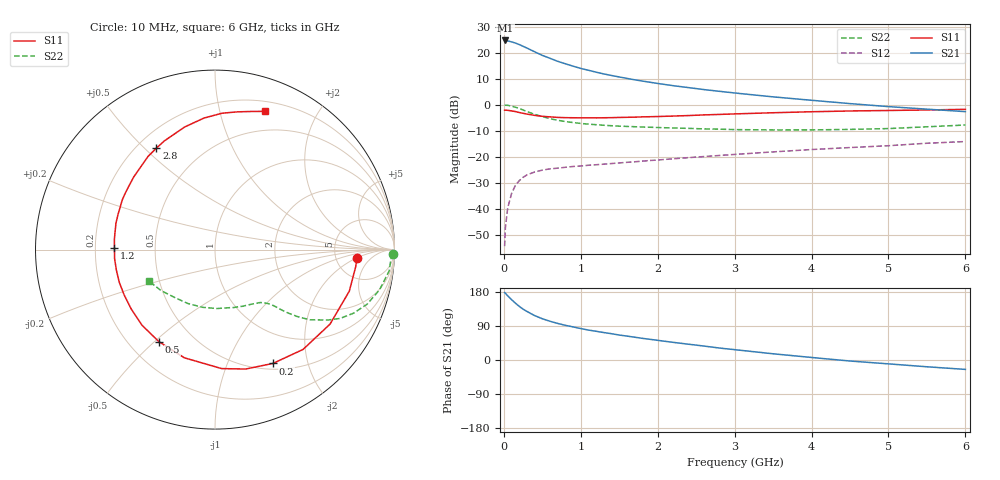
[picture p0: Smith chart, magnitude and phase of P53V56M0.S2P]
! SIEMENS Small Signal Semiconductors
! BFP183
! Si NPN RF Bipolar Junction Transistor in SOT143
! VCE = 3.5 V  IC = 6 mA
! Common Emitter S-Parameters:  March  1996
# GHz  S  MA  R  50
!  f  S11  S21  S12  S22
! GHz  MAG  ANG  MAG  ANG  MAG  ANG  MAG  ANG
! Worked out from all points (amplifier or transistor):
!   36 points, 10 MHz to 6 GHz, reference 50 ohm
!   highest |S21| = 24.8 dB at 20 MHz (marker M1)
!   |S21| within 3 dB of that: start of sweep to 305.8 MHz
!   unconditionally stable (mu >= 1): 1.468 GHz to 5.659 GHz
!   at 250 MHz: K = 0.23, MSG = 25.2 dB, |S12| = -27.9 dB
!   at 1.4 GHz: K = 0.98, MSG = 17.0 dB, |S12| = -22.6 dB
!   at 6 GHz: K = 0.95, MSG = 5.8 dB, |S12| = -14.1 dB
!   lowest NFmin = 1.20 dB at 450 MHz
!   S11 on the Smith chart (normalised r, x): 10 MHz: 8.08, -2.03; 200 MHz: 0.57, -1.47; 500 MHz: 0.32, -0.52; 1.2 GHz: 0.28, +0.01; 2.8 GHz: 0.28, +0.54; 6 GHz: 0.30, +1.38
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0.01  0.7917 -3.4  17.2 178.0  0.0019 86.7  0.9921 -1.4
0.02  0.79 -6.8  17.34 176.1  0.0043 87.7  0.9821 -2.8
0.05  0.7833 -17.2  16.98 169.4  0.0103 84.5  0.9776 -7.0
0.1  0.7637 -32.9  16.3 159.4  0.0195 73.0  0.9434 -13.8
0.15  0.7416 -48.6  15.46 150.0  0.0282 66.0  0.8999 -19.8
0.2  0.7116 -63.0  14.48 141.6  0.0346 59.9  0.8487 -24.7
0.25  0.6871 -75.6  13.38 134.2  0.0402 54.9  0.7959 -28.8
0.3  0.664 -86.8  12.39 128.2  0.0447 51.0  0.7422 -31.9
0.4  0.6265 -105.8  10.49 117.2  0.0509 44.4  0.6578 -36.5
0.5  0.6007 -121.3  8.947 108.9  0.0553 40.1  0.5916 -39.1
0.6  0.5857 -133.9  7.859 102.2  0.0585 37.6  0.5407 -40.9
0.7  0.5722 -144.6  6.878 96.5  0.0603 36.1  0.5034 -42.1
0.9  0.5637 -161.2  5.548 87.3  0.065 33.9  0.4554 -43.6
1.1  0.5617 -174.8  4.622 79.0  0.0687 33.2  0.4244 -45.3
1.2  0.5603 179.2  4.247 75.8  0.0702 33.2  0.4142 -46.2
1.7  0.5789 155.9  3.03 60.2  0.08 34.2  0.3789 -52.1
2.2  0.6074 138.2  2.338 46.6  0.0914 34.7  0.3579 -59.8
2.8  0.6529 120.0  1.821 31.6  0.1057 33.9  0.3399 -71.7
3.5  0.7037 103.9  1.422 16.4  0.1241 32.1  0.3286 -88.2
4.5  0.761 87.0  1.055 -2.7  0.1504 27.1  0.3362 -116.7
5.5  0.796 75.2  0.825 -17.9  0.1821 21.7  0.3774 -142.8
6  0.8185 70.2  0.739 -24.8  0.1962 17.6  0.4086 -154.7
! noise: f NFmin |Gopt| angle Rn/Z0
0.45  1.2  0.21  41  0.24
0.9  1.25  0.24  101  0.21
1.8  2  0.32  175  0.14
